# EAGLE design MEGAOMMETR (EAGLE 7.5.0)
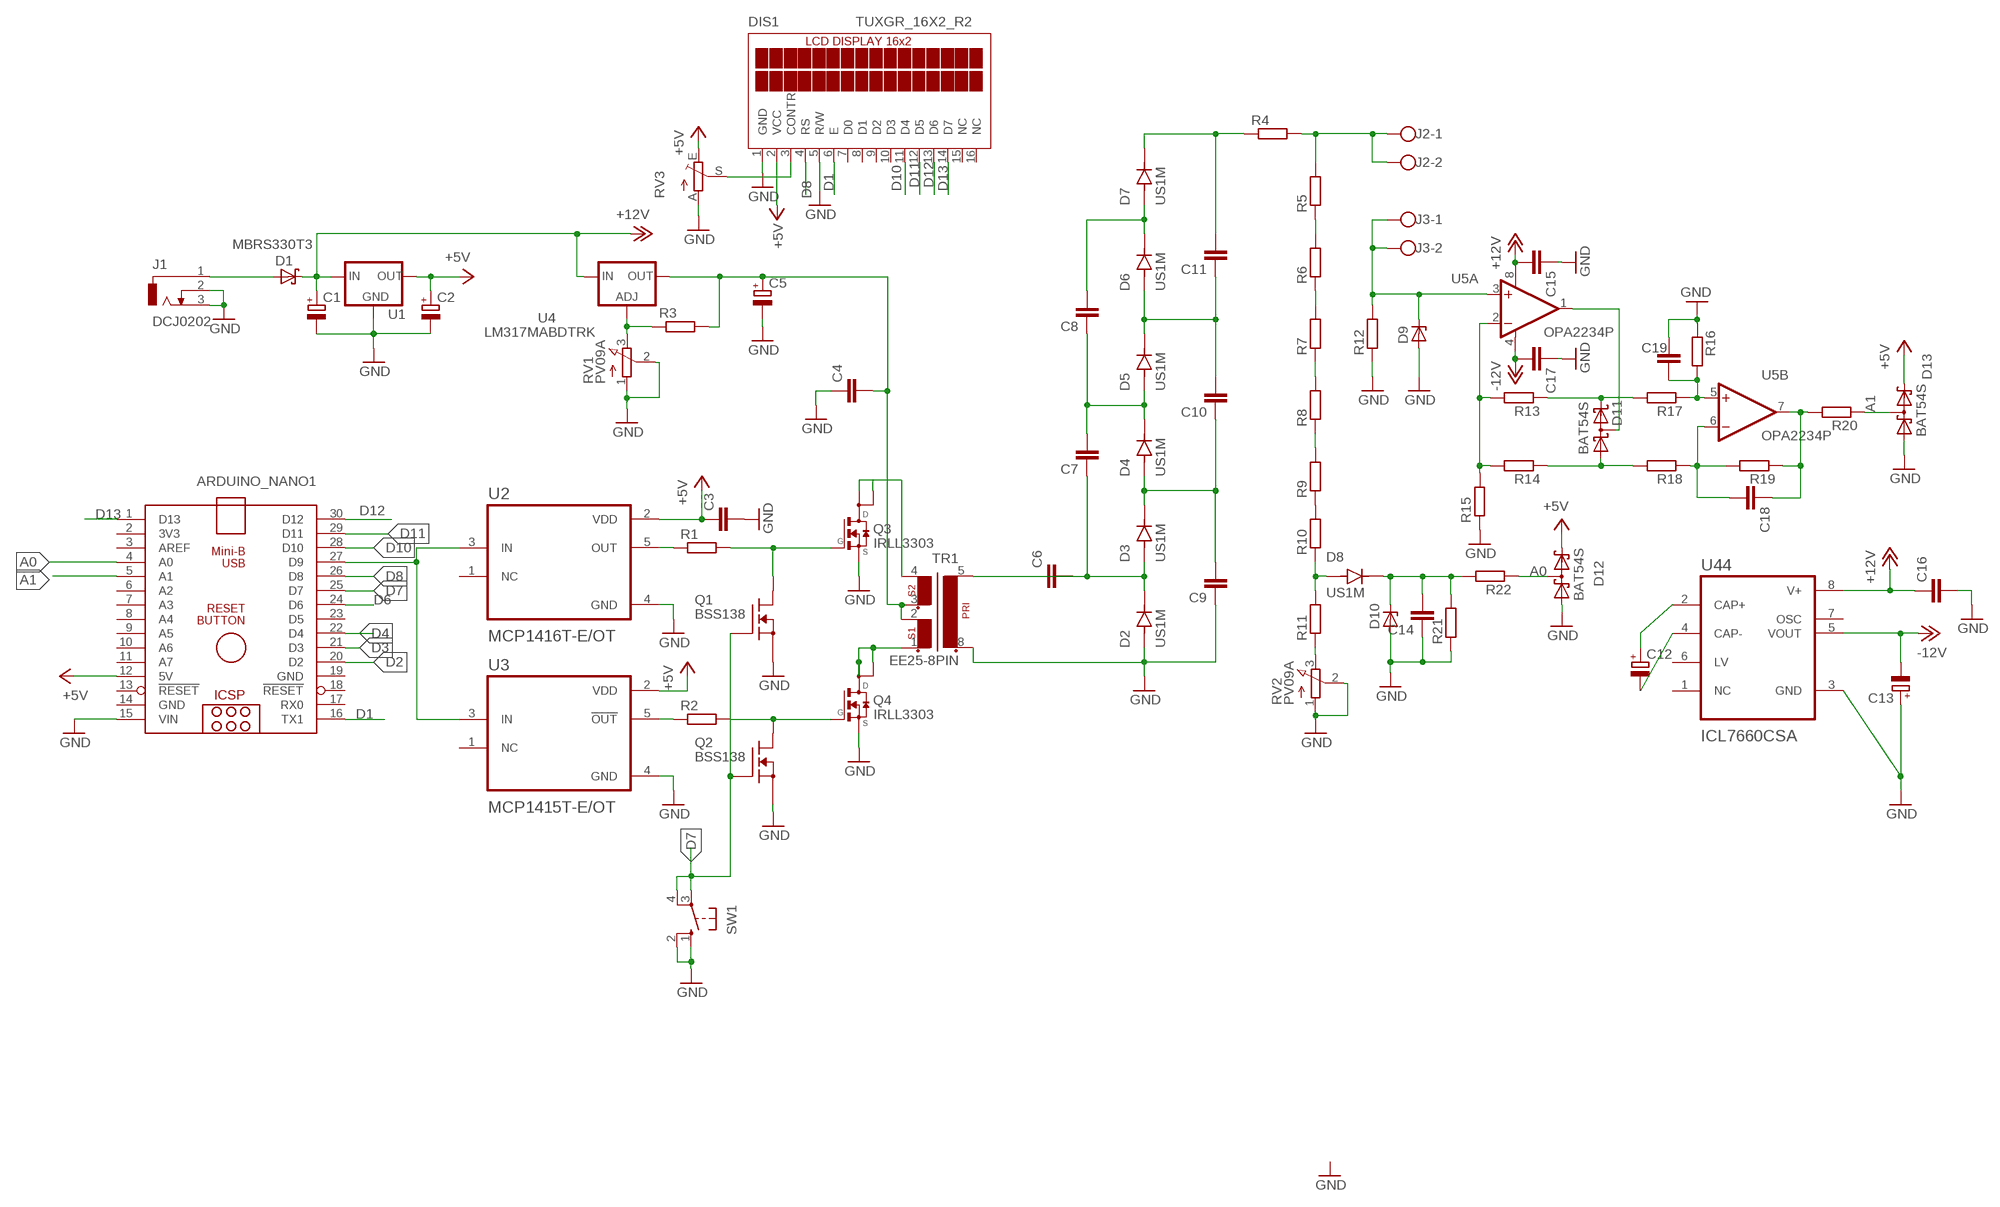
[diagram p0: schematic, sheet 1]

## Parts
ARDUINO_NANO1  ARDUINO_NANO  [ARDUINO_NANO]
C1  CPOL-EUSMCB  [SMC_B]
C2  CPOL-EUSMCB  [SMC_B]
C3  C-EUC1206  [C1206]
C4  C-EUC1206  [C1206]
C5  CPOL-EUSMCE  [SMC_E]
C6  C-EU102-043X133  [C102-043X133]
C7  C-EU102-043X133  [C102-043X133]
C8  C-EU102-043X133  [C102-043X133]
C9  C-EU102-043X133  [C102-043X133]
C10  C-EU102-043X133  [C102-043X133]
C11  C-EU102-043X133  [C102-043X133]
C12  CPOL-EUSMCB  [SMC_B]
C13  CPOL-EUSMCB  [SMC_B]
C14  C-EUC1206  [C1206]
C15  C-EUC1206  [C1206]
C16  C-EUC1206  [C1206]
C17  C-EUC1206  [C1206]
C18  C-EUC1206  [C1206]
C19  C-EUC1206  [C1206]
D1  MBRS330T3  [SMC]
D2  US1M  [DIOM4325X250N]
D3  US1M  [DIOM4325X250N]
D4  US1M  [DIOM4325X250N]
D5  US1M  [DIOM4325X250N]
D6  US1M  [DIOM4325X250N]
D7  US1M  [DIOM4325X250N]
D8  US1M  [DIOM4325X250N]
D9  ZENER-DIODESMB  [SMB]
D10  ZENER-DIODESMB  [SMB]
D11  BAT54S  [SOT23]
D12  BAT54S  [SOT23]
D13  BAT54S  [SOT23]
DIS1  TUXGR_16X2_R2  [TUXGR_16X2_R2]
J1  DCJ0202  [DCJ0202]
J2  W237-102  [W237-102]
J3  W237-102  [W237-102]
Q1  BSS138  [SOT23]
Q2  BSS138  [SOT23]
Q3  IRLL3303  NTF3055L108  [SOT223]
Q4  IRLL3303  NTF3055L108  [SOT223]
R1  R-EU_R1206  [R1206]
R2  R-EU_R1206  [R1206]
R3  R-EU_R1206  [R1206]
R4  R-EU_0207/10  [0207/10]
R5  R-EU_0207/10  [0207/10]
R6  R-EU_0207/10  [0207/10]
R7  R-EU_0207/10  [0207/10]
R8  R-EU_0207/10  [0207/10]
R9  R-EU_0207/10  [0207/10]
R10  R-EU_0207/10  [0207/10]
R11  R-EU_0207/10  [0207/10]
R12  R-EU_R1206  [R1206]
R13  R-EU_R1206  [R1206]
R14  R-EU_R1206  [R1206]
R15  R-EU_R1206  [R1206]
R16  R-EU_R1206  [R1206]
R17  R-EU_R1206  [R1206]
R18  R-EU_R1206  [R1206]
R19  R-EU_R1206  [R1206]
R20  R-EU_R1206  [R1206]
R21  R-EU_R1206  [R1206]
R22  R-EU_R1206  [R1206]
RV1  PV09A  [PTV09]
RV2  PV09A  [PTV09]
RV3  TRIM_EU-B25P  [B25P]
SW1  40-XX  [B3F-40XX]
TR1  EE25-8PIN  EE55-8PIN  [E55-8PIN]
U1  78XXL  [78XXL]
U2  MCP1416T-E/OT  [SOT95P270X145-5N]
U3  MCP1415T-E/OT  [SOT95P270X145-5N]
U4  LM317MABDTRK  [DPACK]
U5  OPA2234P  [DIL08]
U44  ICL7660CSA  [SOIC127P600X175-8N]

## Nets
+5V: ARDUINO_NANO1.12(5V) C2.+ C3.1 D12.2(C2) D13.2(C2) DIS1.2(VCC) RV3.E U1.OUT U2.2(VDD) U3.2(VDD)
+12V: C1.+ C15.2 C16.1 D1.C U1.IN U4.3(IN) U5.8(A:V+) U44.8(V+)
-12V: C13.- C17.2 U5.4(A:V-) U44.5(VOUT)
A0: ARDUINO_NANO1.4(A0) D12.3(C1A2) R22.1
A1: ARDUINO_NANO1.5(A1) D13.3(C1A2) R20.1
D1: ARDUINO_NANO1.16(TX1) DIS1.6(E)
D2: ARDUINO_NANO1.20(D2)
D3: ARDUINO_NANO1.21(D3)
D4: ARDUINO_NANO1.22(D4)
D6: ARDUINO_NANO1.24(D6)
D7: ARDUINO_NANO1.25(D7) Q1.3(G) Q2.3(G) SW1.3(P) SW1.4(P1)
D8: ARDUINO_NANO1.26(D8) DIS1.4(RS)
D10: ARDUINO_NANO1.28(D10) DIS1.11(D4)
D11: ARDUINO_NANO1.29(D11) DIS1.12(D5)
D12: ARDUINO_NANO1.30(D12) DIS1.13(D6)
D13: ARDUINO_NANO1.1(D13) DIS1.14(D7)
GND: ARDUINO_NANO1.15(VIN) C1.- C2.- C3.2 C4.1 C5.- C9.1 C13.+ C14.1 C15.1 C16.2 C17.1 C19.1 D2.A D9.A D10.A D12.1(A1) D13.1(A1) DIS1.1(GND) DIS1.5(R/W) J1.2 J1.3 Q1.1(S) Q2.1(S) Q3.3(S) Q4.3(S) R12.1 R15.1 R16.1 R21.1 RV1.1(A) RV1.2(S) RV2.1(A) RV2.2(S) RV3.A SW1.1(S) SW1.2(S1) TR1.8 U1.GND U2.4(GND) U3.4(GND) U44.3(GND)
N$1: R1.1 U2.5(OUT)
N$2: Q1.2(D) Q3.1(G) R1.2
N$3: R2.1 U3.5(!OUT)
N$4: Q2.2(D) Q4.1(G) R2.2
N$5: ARDUINO_NANO1.27(D9) U2.3(IN) U3.3(IN)
N$6: Q3.2(D) Q3.4(D2) TR1.4
N$7: Q4.2(D) Q4.4(D2) TR1.1
N$8: R3.1 RV1.3(E) U4.1(ADJ)
N$9: C4.2 C5.+ R3.2 TR1.2 TR1.3 U4.4(OUT)
N$10: C6.1 C7.1 D2.C(K) D3.A
N$11: C9.2 C10.1 D3.C(K) D4.A
N$12: C7.2 C8.1 D4.C(K) D5.A
N$13: C10.2 C11.1 D5.C(K) D6.A
N$14: C8.2 D6.C(K) D7.A
N$15: C6.2 TR1.5
N$16: C11.2 D7.C(K) R4.1
N$17: J2.1 J2.2 R4.2 R5.2
N$18: R5.1 R6.2
N$19: R6.1 R7.2
N$20: R7.1 R8.2
N$21: R8.1 R9.2
N$22: R9.1 R10.2
N$23: D9.C J3.1 J3.2 R12.2 U5.3(A:+IN)
N$24: D8.A R10.1 R11.2
N$25: R13.2 R14.2 R15.2 U5.2(A:-IN)
N$26: D11.3(C1A2) U5.1(A:OUT)
N$27: D11.2(C2) R13.1 R17.2
N$28: C12.+ U44.2(CAP+)
N$29: C12.- U44.4(CAP-)
N$30: D11.1(A1) R14.1 R18.2
N$31: C18.2 R18.1 R19.2 U5.6(B:-IN)
N$32: C19.2 R16.2 R17.1 U5.5(B:+IN)
N$33: R11.1 RV2.3(E)
N$35: C14.2 D8.C(K) D10.C R21.2 R22.2
N$36: DIS1.3(CONTR) RV3.S
N$38: C18.1 R19.1 R20.2 U5.7(B:OUT)
N$40: D1.A J1.1
Unconnected: ARDUINO_NANO1.2(3V3) ARDUINO_NANO1.3(AREF) ARDUINO_NANO1.6(A2) ARDUINO_NANO1.7(A3) ARDUINO_NANO1.8(A4) ARDUINO_NANO1.9(A5) ARDUINO_NANO1.10(A6) ARDUINO_NANO1.11(A7) ARDUINO_NANO1.13(!RESET) ARDUINO_NANO1.17(RX0) ARDUINO_NANO1.18(!RESET) ARDUINO_NANO1.23(D5) DIS1.7(D0) DIS1.8(D1) DIS1.9(D2) DIS1.10(D3) DIS1.15(NC) DIS1.16(NC) U2.1(NC) U3.1(NC) U44.1(NC) U44.6(LV) U44.7(OSC)

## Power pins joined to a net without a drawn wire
GND: ARDUINO_NANO1.14(GND) ARDUINO_NANO1.19(GND)

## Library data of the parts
ARDUINO_NANO1 = ArduinoNanoV30:ARDUINO_NANO: Arduino Nano V3.0 Overview: The Arduino Nano is a small, complete, and breadboard-friendly board based on the ATmega328 (Arduino Nano 3.x) or ATmega168 (Arduino Nano 2.x). It has more or less the same functionality of the Arduino Duemilanove, but in a different package. It lacks only a DC power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
C1 C2 C5 C12 C13 = rcl:CPOL-EU: POLARIZED CAPACITOR, European symbol
C3 C4 C6-C11 C14-C19 = rcl:C-EU: CAPACITOR, European symbol
D1 = diode:MBRS3*0T3: SCHOTTKY BARRIER RECTIFIER 3.0 AMPERES 20, 30, 40 VOLT
D2-D8 = US1M:US1M: Check availability; AVAILABILITY: In Stock; CHECK_PRICES: https://www.snapeda.com/parts/US1M/Taiwan+Semiconductor/view-part/?ref=eda; DESCRIPTION: 75ns, 1A, 1000V, High Efficient Recovery Rectifier; MF: Taiwan Semiconductor; MP: US1M; PACKAGE: SMA-2 Taiwan Semiconductor; PRICE: None; SNAPEDA_LINK: https://www.snapeda.com/parts/US1M/Taiwan+Semiconductor/view-part/?ref=snap
D9 D10 = diode:ZENER-DIODE: Z-Diode
D11-D13 = diode:BAT54S: Schottky Diodes Pin connection corrected 2011-05-04 Source: Fairchild .. BAT54.pdf
DIS1 = display-lcd:TUXGR_16X2_R2: Tuxgraphics LCD display 16x2 characters reflective, without background light Source: tuxgr_12x2_r2.pdf; OC_FARNELL: unknown; OC_NEWARK: unknown
J1 = con-jack:DCJ0202: DC POWER JACK Source: DCJ0202.pdf; OC_FARNELL: unknown; OC_NEWARK: unknown
J2 J3 = con-wago-500:W237-102: WAGO SCREW CLAMP; MPN: 237-102; OC_FARNELL: unknown; OC_NEWARK: 70K9898
Q1 Q2 = transistor-fet:BSS138
Q3 Q4 = NTF3055L108:NTF3055L108: N-Channel MOSFET 3.0 A, 60 V Check availability; AVAILABILITY: In Stock; CHECK_PRICES: https://www.snapeda.com/parts/NTF3055L108/Onsemi/view-part/?ref=eda; DESCRIPTION: N-Channel 60 V 3A (Ta) 1.3W (Ta) Surface Mount SOT-223 (TO-261); MF: ON Semiconductor; MP: NTF3055L108; PACKAGE: TO-261-4 ON Semiconductor; PRICE: None; PURCHASE-URL: https://www.snapeda.com/api/url_track_click_mouser/?unipart_id=2731930&manufacturer=ON Semiconductor&part_name=NTF3055L108&search_term=ntf3055; SNAPEDA_LINK: https://www.snapeda.com/parts/NTF3055L108/Onsemi/view-part/?ref=snap
R1-R22 = rcl:R-EU_: RESISTOR, European symbol
RV1 RV2 = pot:PV09A
RV3 = pot:TRIM_EU-: POTENTIOMETER
SW1 = switch-omron:40-XX: OMRON SWITCH; MF: OMRON COMPONENTS USA; MPN: B3F-4000; OC_FARNELL: 176434; OC_NEWARK: 36K3105
TR1 = trafo:EE55-8PIN
U1 = v-reg:78XXL: VOLTAGE REGULATOR
U2 = MCP1416T-E_OT:MCP1416T-E/OT: Check availability; AVAILABILITY: In Stock; CHECK_PRICES: https://www.snapeda.com/parts/MCP1416T-E/OT/Microchip/view-part/?ref=eda; DESCRIPTION: MCP1416T-E/OT,MOSFET Power Driver 1.5A,4.5 to 18V,Non-Inverting,5-Pin SOT-23 | Microchip Technology Inc. MCP1416T-E/OT; MF: Microchip; MP: MCP1416T-E/OT; PACKAGE: SOT-23-5 Microchip; PRICE: None; SNAPEDA_LINK: https://www.snapeda.com/parts/MCP1416T-E/OT/Microchip/view-part/?ref=snap
U3 = MCP1415T-E_OT:MCP1415T-E/OT: Check availability; AVAILABILITY: In Stock; CHECK_PRICES: https://www.snapeda.com/parts/MCP1415T-E/OT/Microchip/view-part/?ref=eda; DESCRIPTION: MCP1415T-E/OT,MOSFET Power Driver 1.5A,4.5 to 18V,Inverting,5-Pin SOT-23 | Microchip Technology Inc. MCP1415T-E/OT; MF: Microchip; MP: MCP1415T-E/OT; PACKAGE: SOT-23-5 Microchip; PRICE: None; SNAPEDA_LINK: https://www.snapeda.com/parts/MCP1415T-E/OT/Microchip/view-part/?ref=snap
U4 = v-reg:LM317?*: 500 mA Adjustable Output Positive Voltage Regulator Source: http://www.onsemi.co.jp .. LM317M-D.PDF
U5 = burr-brown:OPA2234: Operational Amplifier; OC_FARNELL: unknown; OC_NEWARK: unknown
U44 = ICL7660CSA:ICL7660CSA: Check availability; AVAILABILITY: In Stock; CHECK_PRICES: https://www.snapeda.com/parts/ICL7660CSA/Analog+Devices/view-part/?ref=eda; DESCRIPTION: Charge Pump Switching Regulator IC Positive or Negative Fixed -Vin, nVin, Vin/2 1 Output 20mA 8-SOIC (0.154, 3.90mm Width); MF: Analog Devices; MP: ICL7660CSA; PACKAGE: SOIC-8 Maxim; PRICE: None; SNAPEDA_LINK: https://www.snapeda.com/parts/ICL7660CSA/Analog+Devices/view-part/?ref=snap

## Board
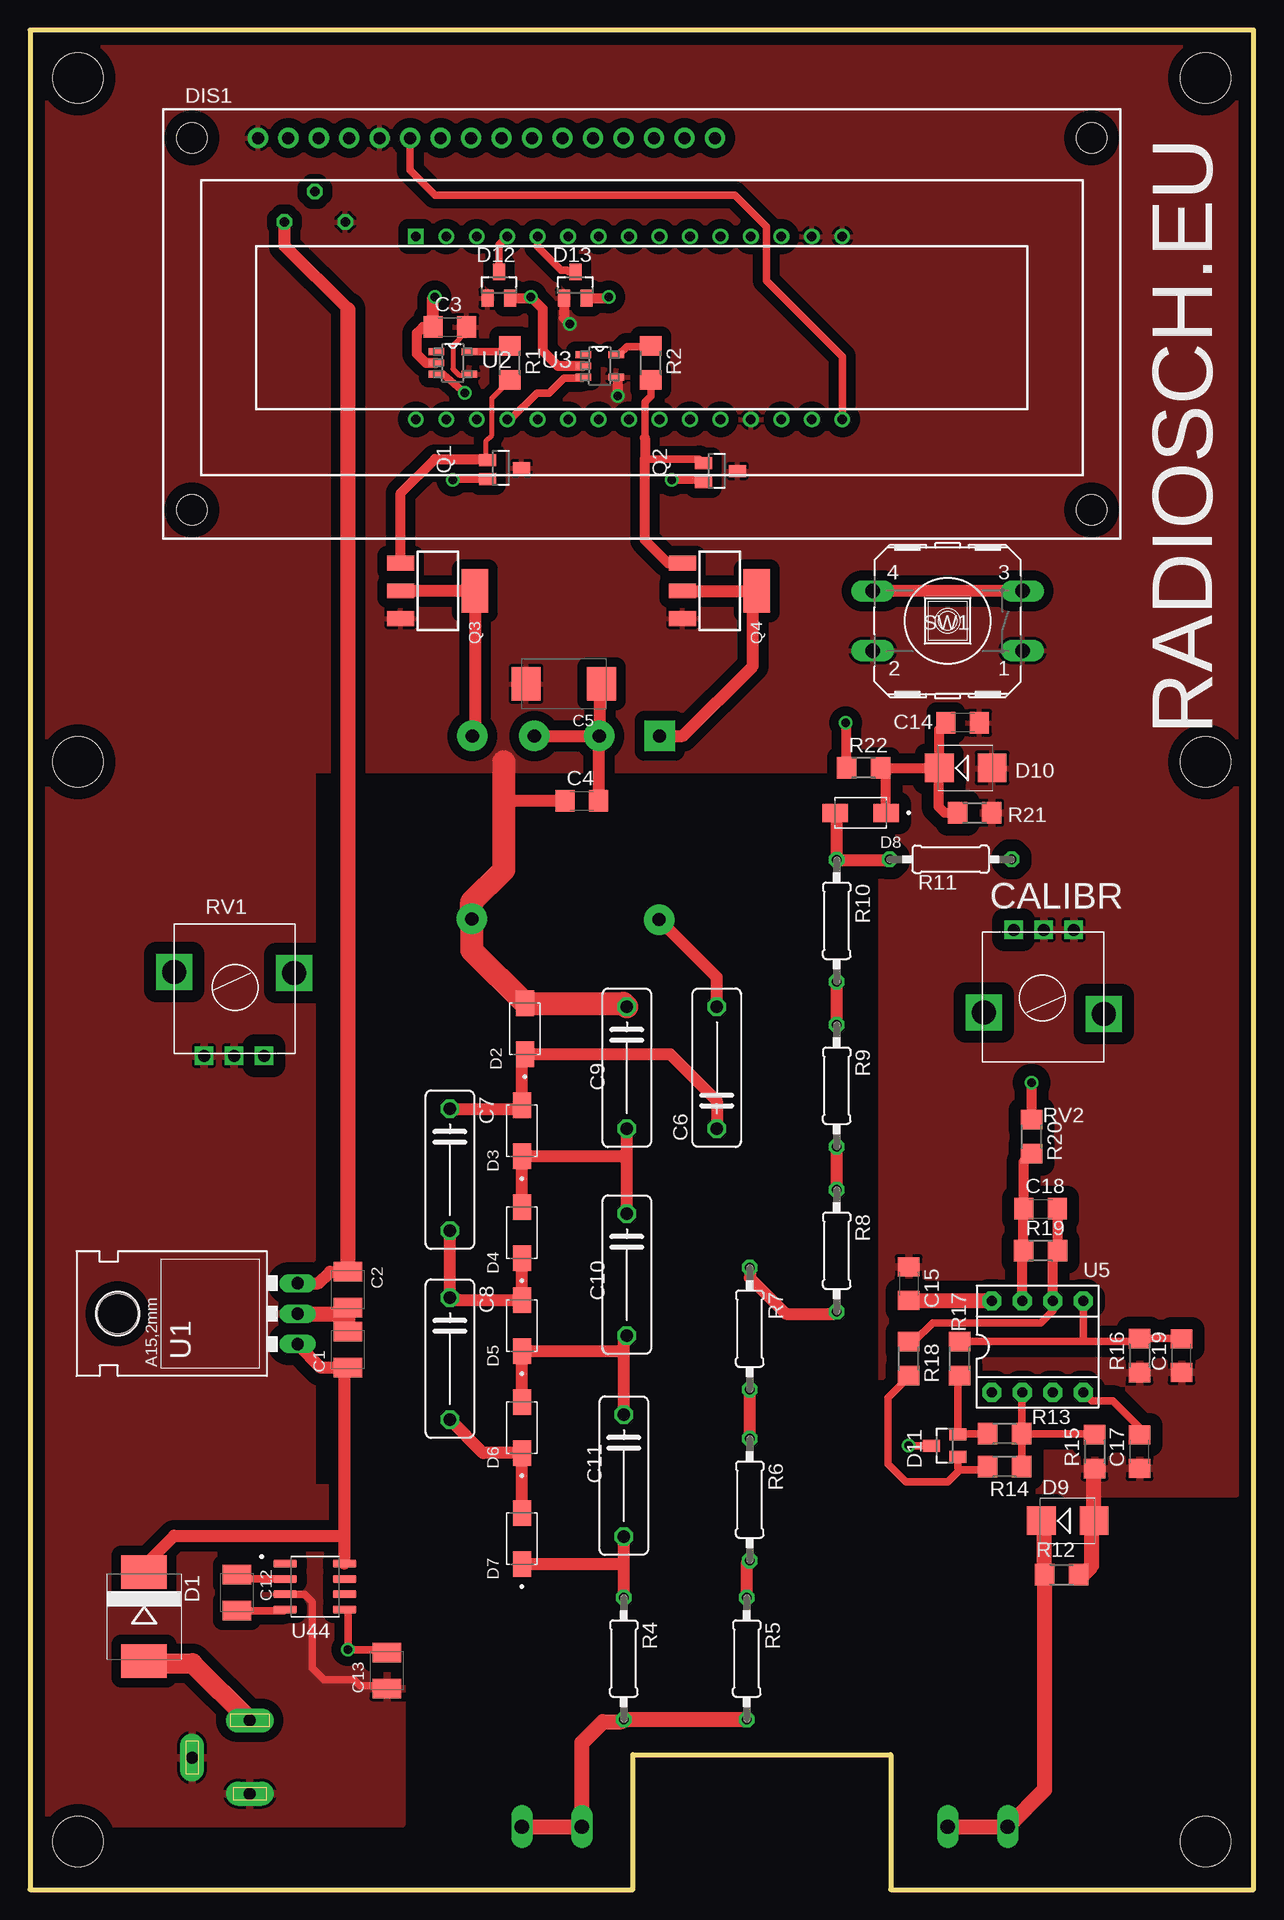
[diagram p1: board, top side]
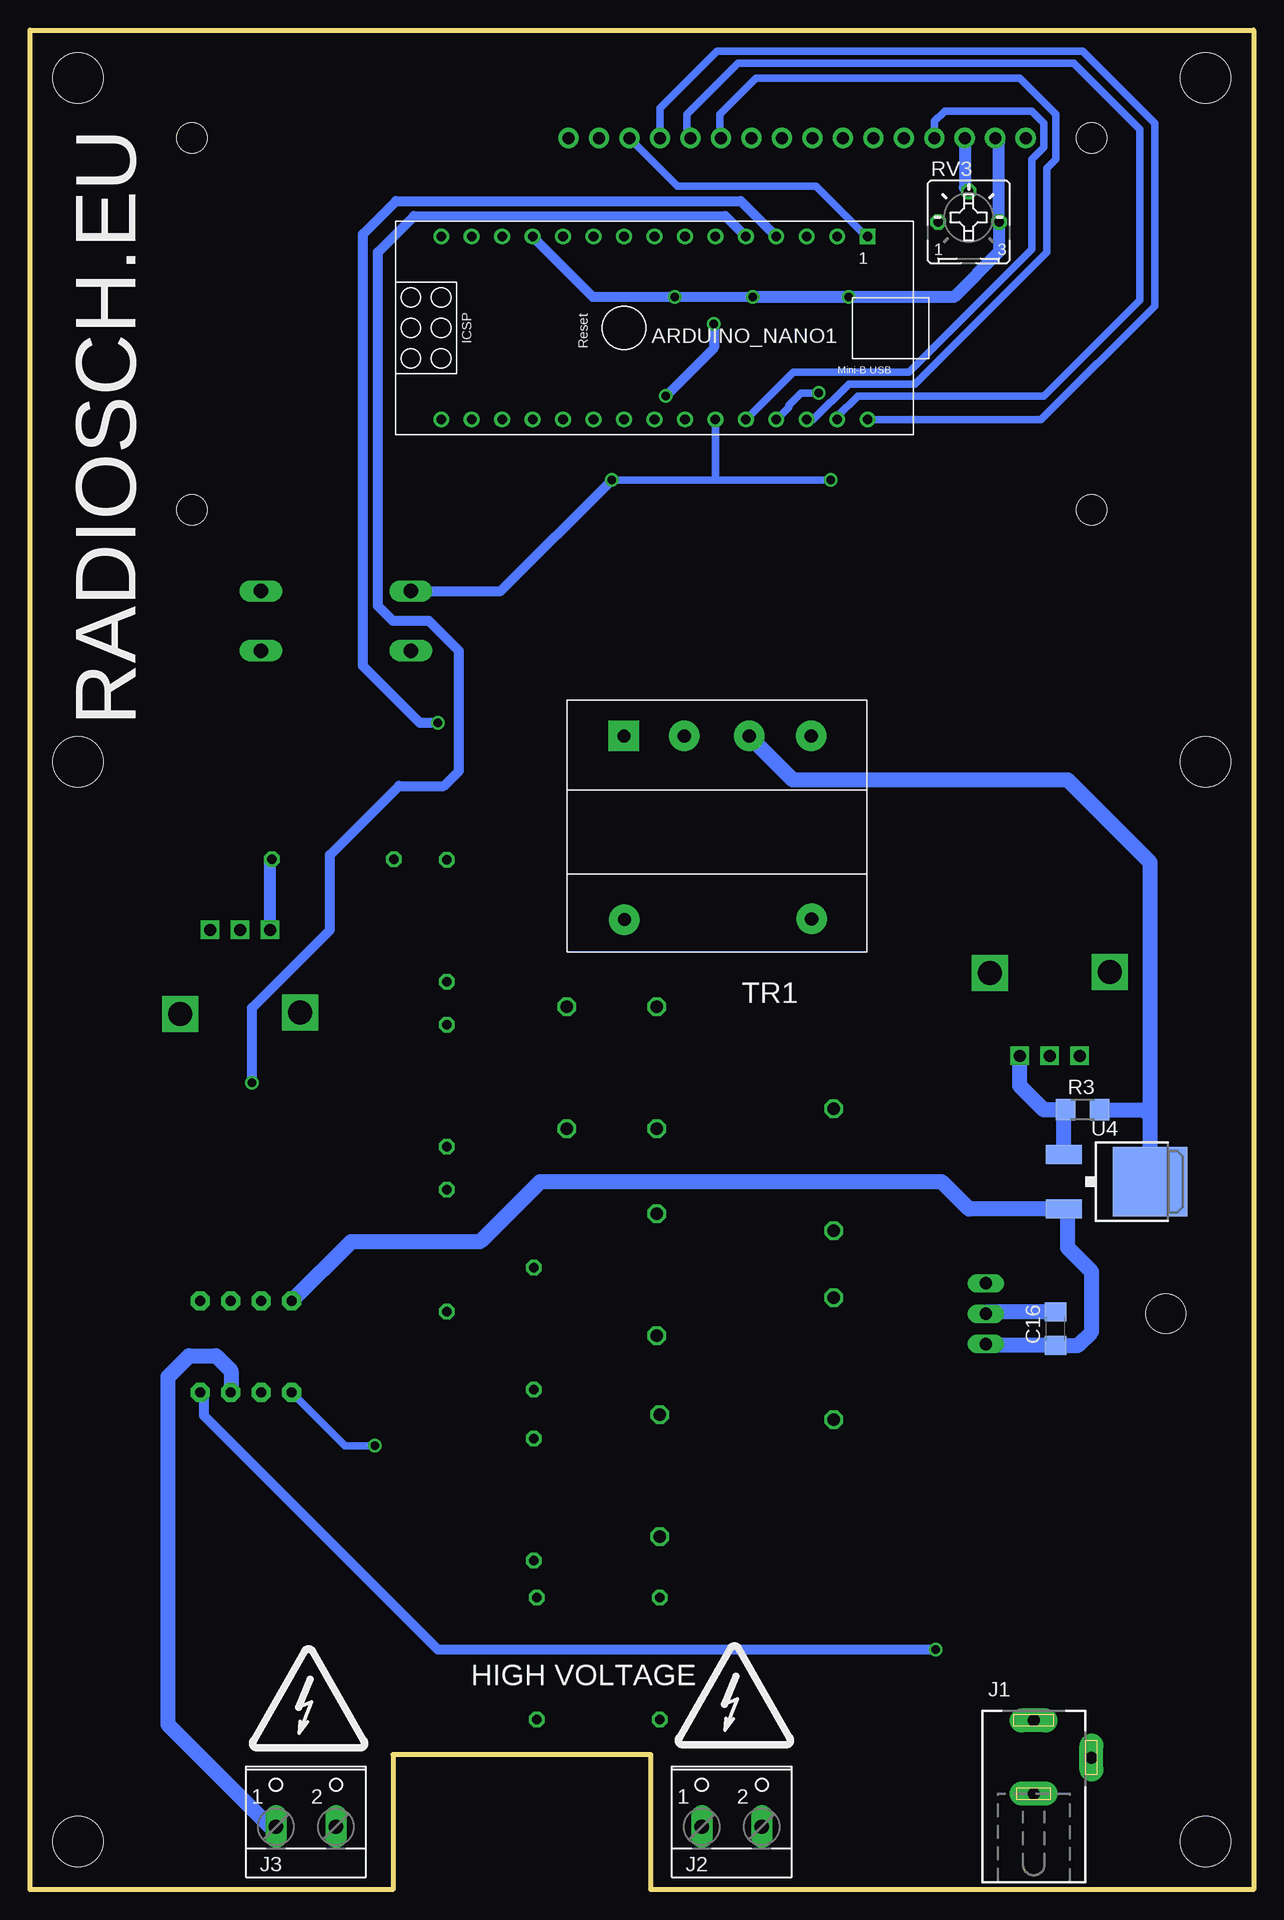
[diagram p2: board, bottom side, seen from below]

Size 102 x 155 mm. Coordinates in mm from the lower left corner, seen from the top.
Outline: 0,0 50.25,0 50.25,11.25 71.75,11.25 71.75,0 102,0 102,155 0,155 0,0
Copper layers (1*16): Top 0.035mm / dielectric 1.5mm / Bottom 0.035mm
Design rules "default": minimum track width 10mil, minimum drill 24mil, track to track 8mil, track to pad 8mil, pad to pad 8mil, via to via 8mil, smd to smd 8mil, copper to edge 40mil, drill to drill 8mil, minimum pad ring 10mil, minimum via ring 8mil, stop-mask expansion 4mil, vias tented up to drill 0mil, thermal gap 10mil
Holes 4.2 mm at 4,151 98,151 4,4 98,4 4,94 98,94

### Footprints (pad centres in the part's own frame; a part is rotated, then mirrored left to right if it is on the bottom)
ARDUINO_NANO = drill 0.8 square: 1 -20.32,-7.62 | drill 0.8: 2 -17.78,-7.62; 3 -15.24,-7.62; 4 -12.7,-7.62; 5 -10.16,-7.62; 6 -7.62,-7.62; 7 -5.08,-7.62; 8 -2.54,-7.62; 9 0,-7.62; 10 2.54,-7.62; 11 5.08,-7.62; 12 7.62,-7.62; 13 10.16,-7.62; 14 12.7,-7.62; 15 15.24,-7.62; 16 15.24,7.62; 17 12.7,7.62; 18 10.16,7.62; 19 7.62,7.62; 20 5.08,7.62; 21 2.54,7.62; 22 0,7.62; 23 -2.54,7.62; 24 -5.08,7.62; 25 -7.62,7.62; 26 -10.16,7.62; 27 -12.7,7.62; 28 -15.24,7.62; 29 -17.78,7.62; 30 -20.32,7.62
SMC_B = smd 1.6 x 2.4: + -1.5,0; - 1.5,0
C1206 = smd 1.6 x 1.8: 1 -1.4,0; 2 1.4,0
SMC_E = smd 2.4 x 2.8: + -3.15,0; - 3.15,0
C102-043X133 = drill 1.016 octagon: 1 -5.08,0; 2 5.08,0
SMC = smd 2.8 x 3.8: A 3.7,0; C -3.7,0
DIOM4325X250N = smd 2.12 x 1.5: A 2.115,0; C -2.115,0
SMB = smd 2.4 x 2.4: A 2.2,0; C -2.2,0
SOT23 = smd 1 x 1.4: 1 -0.95,-1.1; 2 0.95,-1.1; 3 0,1.1
TUXGR_16X2_R2 = drill 1 pad 1.676: 1 -32,15.5; 2 -29.46,15.5; 3 -26.92,15.5; 4 -24.38,15.5; 5 -21.84,15.5; 6 -19.3,15.5; 7 -16.76,15.5; 8 -14.22,15.5; 9 -11.68,15.5; 10 -9.14,15.5; 11 -6.6,15.5; 12 -4.06,15.5; 13 -1.52,15.5; 14 1.02,15.5; 15 3.56,15.5; 16 6.1,15.5 | hole 2.5: -37.5,-15.5; 37.5,-15.5; -37.5,15.5; 37.5,15.5
DCJ0202 = drill 1 pad 2 long: 1 0,3.1; 2 4.8,0; 3 0,-3
W237-102 = drill 1.194 long: 1 -2.5,-1.27; 2 2.5,-1.27
SOT23' = smd 1 x 1.4: 1 0,1.735; 2 -0.632,-1.1; 3 0.95,-1.1
SOT223 = smd 1.219 x 2.235: 1 -2.311,-3.099; 2 0,-3.099; 3 2.311,-3.099 | smd 3.6 x 2.2: 4 0,3.099
R1206 = smd 1.6 x 1.803: 1 -1.422,0; 2 1.422,0
0207/10 = drill 0.813 octagon: 1 -5.08,0; 2 5.08,0
PTV09 = drill 1 square: 1 -2.5,0; 2 0,0; 3 2.5,0 | drill 2 square: P$4 -5,7; P$5 5,6.9
B25P = drill 0.813 octagon: A -2.54,0; E 2.54,0; S 0,2.54
B3F-40XX = drill 1.194 long: 1 -6.248,2.489; 2 6.248,2.489; 3 -6.248,-2.489; 4 6.248,-2.489
E55-8PIN = drill 1.1 pad 2.54 square: 1 21.74,0 | drill 1.1 pad 2.54: 2 11.3,0; 3 16.7,0; 4 6.125,0; 5 21.69,15.3; 8 6.075,15.25
78XXL = drill 1.016 long: GND 0,-3.81; IN -2.54,-3.81; OUT 2.54,-3.81 | hole 3.302: 0,11.176
SOT95P270X145-5N = smd 1.321 x 0.559: 1 -1.372,0.94; 2 -1.372,0; 3 -1.372,-0.94; 4 1.372,-0.94; 5 1.372,0.94
DPACK = smd 1.6 x 3: 1 -2.28,-4.8; 3 2.28,-4.8 | smd 5.8 x 6.2: 4 0,2.38
DIL08 = drill 0.813 pad 1.6 octagon: 1 -3.81,-3.81; 2 -1.27,-3.81; 3 1.27,-3.81; 4 3.81,-3.81; 5 3.81,3.81; 6 1.27,3.81; 7 -1.27,3.81; 8 -3.81,3.81
SOIC127P600X175-8N = smd 1.97 x 0.59: 1 -2.475,1.905; 2 -2.475,0.635; 3 -2.475,-0.635; 4 -2.475,-1.905; 5 2.475,-1.905; 6 2.475,-0.635; 7 2.475,0.635; 8 2.475,1.905

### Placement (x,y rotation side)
ARDUINO_NANO1  52.48,130.16 180 bottom
C1  26.5,45 90 top
C2  26.5,50 270 top
C3  35,130.25 0 top
C4  46,90.75 0 top
C5  44.5,100.5 180 top
C6  57.25,68.5 90 top
C7  35,60 270 top
C8  35,44.25 270 top
C9  49.75,68.5 270 top
C10  49.75,51.25 270 top
C11  49.5,34.5 270 top
C12  17.25,24.75 270 top
C13  29.75,18.25 90 top
C14  77.75,97.25 180 top
C15  73.25,50.5 270 top
C16  16.5,46.75 90 bottom
C17  92.5,36.5 90 top
C18  84.25,56.75 0 top
C19  96,44.5 90 top
D1  9.5,22.75 270 top
D2  41.25,71.75 90 top
D3  41,63.25 90 top
D4  41,54.75 90 top
D5  41,47 90 top
D6  41,38.5 90 top
D7  41,29.25 90 top
D8  69.25,89.75 180 top
D9  86.5,30.75 0 top
D10  78,93.5 0 top
D11  76.25,37 90 top
D12  39.09,133.74 0 top
D13  45.46,133.74 0 top
DIS1  51,130.5 0 top
J1  18.32,10.99 0 bottom
J2  43.5,6.5 0 bottom
J3  79,6.5 0 bottom
Q1  BSS138  [SOT23']  39.25,118.5 270 top
Q2  BSS138  [SOT23']  57.25,118.25 270 top
Q3  34,108.25 270 top
Q4  57.5,108.25 270 top
R1  40,127.25 270 top
R2  51.75,127.25 270 top
R3  14.25,65 0 bottom
R4  49.5,19.25 270 top
R5  59.75,19.25 270 top
R6  60,32.5 270 top
R7  60,46.75 270 top
R8  67.25,53.25 270 top
R9  67.25,67 270 top
R10  67.25,80.75 270 top
R11  76.75,85.88 180 top
R12  86,26.25 180 top
R13  81.25,38 0 top
R14  81.25,35.25 0 top
R15  88.75,36.5 90 top
R16  92.5,44.5 90 top
R17  77.5,44.25 270 top
R18  73.25,44.25 270 top
R19  84.25,53.25 0 top
R20  83.5,62.75 270 top
R21  78.75,89.75 180 top
R22  69.5,93.5 0 top
RV1  17,69.5 0 top
RV2  84.5,80 180 top
RV3  23.75,139 0 bottom
SW1  76.5,105.75 180 top
TR1  30.75,96.15 180 bottom
U1  18.5,48 90 top
U2  35.25,127.25 0 top
U3  47.5,127 0 top
U4  11,59 270 bottom
U5  84,45.25 0 top
U44  23.75,25.25 0 top
U$1  [RADIOACTIVE_10.00]  84,11.5 0 bottom
U$2  [RADIOACTIVE_10.00]  48.5,11.75 0 bottom

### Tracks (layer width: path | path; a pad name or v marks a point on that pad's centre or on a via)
+5V  (via drill 0.7)
  Top 0.813: D12.2 41.64,132.64 v41.75,132.75 42.75,131.75 42.75,128.25 44,127 U3.2 | D13.2 48.14,132.64 v48.25,132.75 | U2.2 33,127.25 32.25,128 32.25,129.75 32.75,130.25 C3.1
  Top 1.016: C3.1 33.6,132.6 v33.75,132.75 | 26.5,131.71 21.21,137 RV3.E | U1.OUT 24.04,50.54 25,51.5 C2.+
  Top 1.27: C2.+ 26.5,131.71
  Bottom 0.813: v41.75,132.75 v48.25,132.75 55.07,132.75 ARDUINO_NANO1.12
  Bottom 1.016: DIS1.2 21.21,145.67 RV3.E 21.21,136.54 25,132.75 v33.75,132.75 v41.75,132.75
+12V
  Top 1.016: U1.IN 24.27,43.5 C1.+ 26.23,43.23 26.23,29.5 | U44.8 26.23,29.5 | D1.C 9.5,27 12,29.5 26.23,29.5
  Top 1.27: C15.2 80.15,49.1 U5.8
  Bottom 1.27: U5.8 75.25,54 64.5,54 59.5,59 26,59 23.72,56.72 U4.3 15.5,56.42 15.5,53.5 13.5,51.5 13.5,46.5 14.65,45.35 C16.1 22.2,45.35 U1.IN
-12V  (via drill 0.7)
  Top 0.61: U44.5 26.5,23.07 v26.5,20 29.5,20 C13.- | C17.2 92.5,38.5 90.25,40.75 88.5,40.75 U5.4
  Bottom 0.813: v26.5,20 68,20 87.5,39.5 87.5,41.13 U5.4
A0  (via drill 0.7)
  Top 0.61: D12.3 39.09,137.09 ARDUINO_NANO1.4
  Top 0.813: R22.1 68.08,97.17 v68,97.25
  Bottom 0.813: v68,97.25 69.5,97.25 74.25,102 74.25,138 71.5,140.75 42.75,140.75 ARDUINO_NANO1.4
A1  (via drill 0.7)
  Top 0.61: D13.3 44.91,134.84 44.75,135 44.25,135 42.32,136.93 ARDUINO_NANO1.5
  Top 0.813: R20.1 v83.5,67.25
  Bottom 0.813: v83.5,67.25 83.5,73.5 77,80 77,86.25 71.25,92 67.5,92 66.25,93.25 66.25,103.25 68.75,105.75 71.75,105.75 73,107 73,136.5 70,139.5 44.04,139.5 ARDUINO_NANO1.5
D1
  Top 0.61: DIS1.6 31.7,143.3 33.75,141.25 58.75,141.25 61.38,138.62 61.38,134.12 67.72,127.78 ARDUINO_NANO1.16
D7  (via drill 0.7)
  Top 0.61: Q1.3 35.3,117.55 v35.25,117.5 | v53.5,117.5 55.5,117.5 55.75,117.25 56.1,117.25 Q2.3
  Top 1.016: SW1.3 SW1.4
  Bottom 0.61: v35.25,117.5 45,117.5 | 45,117.5 v53.5,117.5 | ARDUINO_NANO1.25 44.86,117.64 45,117.5
  Bottom 0.813: SW1.4 62.76,108.24 v53.5,117.5
D8
  Bottom 0.61: DIS1.4 26.62,147.38 25.75,148.25 18.5,148.25 17.5,147.25 17.5,145.25 18.5,144.25 18.5,136.75 28.75,126.5 38.36,126.5 ARDUINO_NANO1.26
D10
  Bottom 0.61: ARDUINO_NANO1.28 36.71,122.54 33.75,125.5 28.25,125.5 17.25,136.5 17.25,143.5 16.5,144.25 16.5,148 19.5,151 41.5,151 44.5,148 44.5,146.1 DIS1.11
D11
  Bottom 0.61: ARDUINO_NANO1.29 34.7,122.8 33,124.5 17.5,124.5 9.5,132.5 9.5,146.75 15,152.25 43,152.25 47.25,148 47.25,146.31 DIS1.12
D12
  Bottom 0.61: ARDUINO_NANO1.30 17.71,122.54 8.25,132 8.25,147.25 14.25,153.25 44.75,153.25 49.5,148.5 49.5,146.02 DIS1.13
D13
  Bottom 0.61: ARDUINO_NANO1.1 32.28,137.78 36.5,142 48.02,142 DIS1.14
GND  (via drill 0.7)
  Top 0.406: C3.2 36.4,129.9 35.25,128.75 35.25,126.75 35.75,126.25 36.56,126.25 U2.4
  Top 0.61: U44.3 22.89,24.62 23.5,24 23.5,18.5 24.5,17.5 27,17.5 27.5,17 29.5,17 C13.+
  Top 0.813: D13.1 44.51,130.99 v45,130.5 | v49,124.5 49,125.93 U3.4
  Top 1.016: C4.1 39.5,90.75 39.5,91.25
  Top 1.27: C1.- 26.5,48 | 26.5,48 C2.- | U1.GND 26.5,48 | R15.1 88.7,35.03 D9.A 88.5,30.55 88.5,27 87.75,26.25 R12.1
  Top 1.93: 39.5,94 39.5,91.25 39.5,85 36.83,82.33 TR1.8 36.83,78.29 D2.A 49.47,73.87 C9.1
  Bottom 0.813: v45,130.5 45,128.5 v49,124.5
  Bottom 1.27: C16.2 22.16,48.15 U1.GND
  pour Top (isolate 0.813): 0.75,153.75 100.5,153.75 100.5,93.25 0.75,93.25
  pour Top (isolate 1.016): 83.88,93.12 100.5,93.12 100.5,33 71,33 71,93 87.5,93
  pour Top (isolate 1.016): 1,93.5 23.5,93.5 23.5,5.5 1,5.5
  pour Top (isolate 0.813): 23.5,5.5 31,5.5 31,33.5 1,33.5 1,5.5
N$1
  Top 0.61: U2.5 39.52,128.19 R1.1
N$2
  Top 0.406: 38.03,119.25 38.03,120.78 38.5,121.25 38.5,124.33 R1.2
  Top 0.813: Q3.1 30.9,116.4 33.75,119.25 38.03,119.25 Q1.2
N$3
  Top 0.61: U3.5 49.06,127.94 49.75,128.62 51.7,128.62 R2.1
N$4
  Top 0.61: R2.2 51.75,124.5 51.25,124 51.25,121 | 51.25,119.25 55.78,119.25 Q2.2
  Top 0.813: 51.25,121 51.25,119.25 51.25,112.5 53.19,110.56 Q4.1
N$5  (via drill 0.7)
  Top 0.61: ARDUINO_NANO1.27 40.04,122.54 42.25,124.75 43.25,124.75 44.5,126 46.07,126 U3.3 | U2.3 34.44,126.31 v36.25,124.75
  Bottom 0.61: v36.25,124.75 37.75,124.75 38.75,123.75 38.75,123.57 ARDUINO_NANO1.27
N$6
  Top 1.016: 37.15,96.43 TR1.4 37.1,96.37 Q3.4 Q3.2
N$7
  Top 1.016: Q4.2 Q4.4 60.25,107.9 60.25,102 54.4,96.15 TR1.1
N$8
  Bottom 1.27: U4.1 15.8,64.87 R3.1 17.5,65 19.5,67 RV1.3
N$9
  Top 1.016: TR1.3 47.5,96.2 47.5,100.35 C5.+ | TR1.2 TR1.3 | C4.2 47.45,90.75 TR1.3
  Bottom 1.27: U4.4 8.62,64.5 | 8.62,64.5 8.62,85.62 15.5,92.5 38.4,92.5 TR1.2 | R3.2 9.12,65 8.62,64.5
N$10
  Top 1.016: C6.1 57.25,65.75 53.37,69.63 D2.C 41,69.38 D3.A 40.72,65.08 C7.1
N$11
  Top 1.016: C10.1 49.75,60.75 | 49.75,60.75 C9.2 | D3.C 41.5,61.13 | 41.5,61.13 49.37,61.13 49.75,60.75 | D4.A 41,60.63 41.5,61.13
N$12
  Top 1.016: C7.2 C8.1 35.22,49.12 D5.A D4.C
N$13
  Top 1.016: C11.1 49.5,45 | 49.5,45 49.5,45.92 C10.2 | D5.C 41.5,44.89 | 41.5,44.89 49.38,44.89 49.5,45 | D6.A 41,44.39 41.5,44.89
N$14
  Top 1.016: D7.A D6.C 37.78,36.39 C8.2
N$15
  Top 1.016: C6.2 57.25,76.04 TR1.5
N$16
  Top 1.016: R4.1 49.5,27.25 | 49.5,27.25 C11.2 | D7.C 49.38,27.13 49.5,27.25
N$17
  Top 1.27: R5.2 R4.2 49.33,14 47.75,14 46,12.25 J2.1 J2.2
N$18
  Top 1.016: R5.1 59.75,27.17 R6.2
N$19
  Top 1.016: R6.1 R7.2
N$20
  Top 1.016: R7.1 60,51 63,48 67.08,48 R8.2
N$21
  Top 1.016: R8.1 R9.2
N$22
  Top 1.016: R9.1 R10.2
N$23
  Top 1.27: D9.C 84.58,30.47 R12.2 84.58,8.31 J3.1 J3.2
  Bottom 1.27: J3.1 81.98,5.23 90.5,13.75 90.5,42.75 88.75,44.5 86.5,44.5 85.25,43.25 85.25,41.46 U5.3
N$24
  Top 1.016: R11.2 71.62,85.83 R10.1 67.25,89.64 D8.A
N$25
  Top 0.61: R14.2 R13.2 | R13.2 82.67,41.38 U5.2 | R13.2 88.67,38 R15.2
N$26  (via drill 0.7)
  Top 0.61: D11.3 v73.25,37
  Bottom 0.61: v73.25,37 75.75,37 U5.1
N$27
  Top 0.61: R17.2 77.35,42.68 D11.2 77.4,38 R13.1
N$28
  Top 0.61: U44.2 17.62,25.88 C12.+
N$29
  Top 0.61: C12.- 21.18,23.25 U44.4
N$30
  Top 0.61: R18.2 73.25,42.75 71.5,41 71.5,35.5 73,34 76.5,34 77.5,35 | 77.5,35 79.58,35 R14.1 | D11.1 77.35,35.15 77.5,35
N$31
  Top 0.61: R18.1 73.67,45.67 75.25,47.25 84.25,47.25 85.25,48.25 85.25,49.04 U5.6
  Top 0.813: U5.6 85.27,52.85 R19.2 85.67,56.73 C18.2
N$32
  Top 0.61: R17.1 87.75,45.67 | 87.75,45.67 92.25,45.67 R16.2 95.98,45.92 C19.2 | U5.5 87.81,45.73 87.75,45.67
N$33
  Bottom 1.016: RV2.3 82,85.7 R11.1
N$35
  Top 0.813: D10.C R22.2 71.36,93.06 D8.C | D10.C 75.8,96.7 C14.2 | R21.2 76.25,89.75 75.75,90.25 75.75,93.45 D10.C
N$36
  Bottom 1.016: DIS1.3 24.08,141.87 RV3.S
N$38
  Top 0.813: U5.7 82.73,53.15 R19.1 82.83,56.73 C18.1 82.85,60.68 R20.2
N$40
  Top 1.27: 9.32,18.87 D1.A
  Top 1.676: 9.32,18.87 13.54,18.87 J1.1

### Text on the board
tPlace: RADIOSCH.EU | CALIBR
bPlace: RADIOSCH.EU | HIGH VOLTAGE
